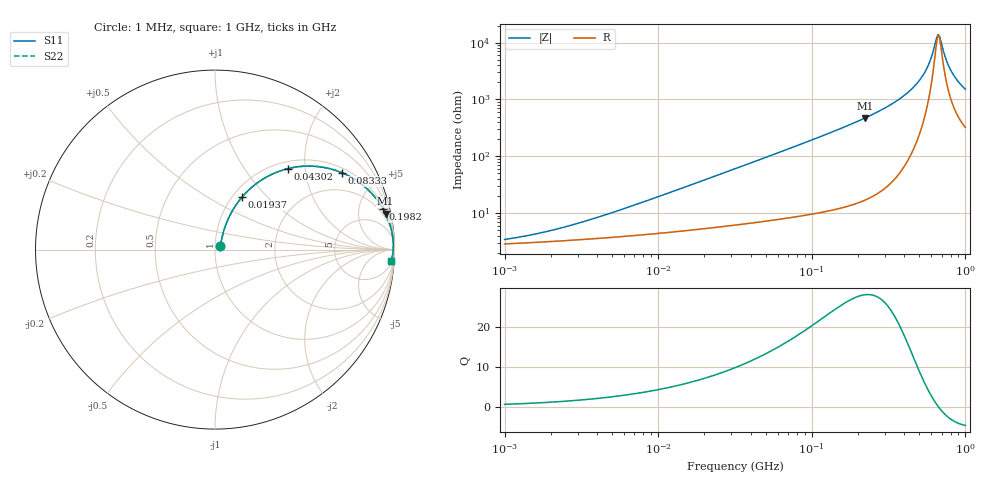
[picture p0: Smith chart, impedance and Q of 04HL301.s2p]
! Coilcraft 0402HL-301 Chip Inductor
! 20 July 2012
# MHz S MA R 50
!Freq  MagS11  AngS11  MagS21  AngS21  MagS12  AngS12  MagS22  AngS22
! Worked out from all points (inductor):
!   304 points, 1 MHz to 1 GHz, reference 50 ohm
!   read as one part in series: L = 300 nH near 6.196 MHz
!   highest Q = 28 at 222.1 MHz (marker M1), where L = 337 nH
!   self-resonance near 663.4 MHz
!   S11 on the Smith chart (normalised r, x): 1 MHz: 1.06, +0.04; 19.37 MHz: 1.10, +0.73; 43.02 MHz: 1.14, +1.63; 83.33 MHz: 1.18, +3.19; 198.2 MHz: 1.30, +8.19; 1 GHz: 7, -29
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1  0.03322 32.4  0.9721 -1.0  0.9721 -1.0  0.03322 32.4
1.768173  0.04401 45.4  0.9696 -1.9  0.9696 -1.9  0.04401 45.4
3.19853  0.06684 57.2  0.9655 -3.3  0.9655 -3.3  0.06684 57.2
10  0.1825 66.7  0.9429 -10.2  0.9429 -10.2  0.1825 66.7
19.36996  0.3314 62.7  0.8977 -19.1  0.8977 -19.1  0.3314 62.7
31.9853  0.4973 54.6  0.8188 -29.7  0.8188 -29.7  0.4973 54.6
43.0193  0.6085 47.9  0.7447 -37.3  0.7447 -37.3  0.6085 47.9
83.32822  0.8275 31.1  0.5179 -55.7  0.5179 -55.7  0.8275 31.1
102.306  0.8753 26.2  0.4427 -61.0  0.4427 -61.0  0.8753 26.2
198.1663  0.9635 13.6  0.235 -74.3  0.235 -74.3  0.9635 13.6
222.0929  0.9712 11.9  0.2062 -76.1  0.2062 -76.1  0.9712 11.9
319.853  0.9869 7.2  0.1261 -80.4  0.1261 -80.4  0.9869 7.2
420.4965  0.9924 4.3  0.07559 -82.1  0.07559 -82.1  0.9924 4.3
516.2633  0.9939 2.4  0.04139 -80.3  0.04139 -80.3  0.9939 2.4
552.8079  0.9939 1.7  0.03054 -77.7  0.03054 -77.7  0.9939 1.7
591.9394  0.9938 1.1  0.02007 -71.3  0.02007 -71.3  0.9938 1.1
663.4103  0.993 0.1  0.007127 -9.5  0.007127 -9.5  0.993 0.1
678.7083  0.9927 -0.1  0.00764 18.0  0.00764 18.0  0.9927 -0.1
743.5105  0.9915 -1.0  0.01862 62.4  0.01862 62.4  0.9915 -1.0
796.1412  0.9903 -1.6  0.02891 69.6  0.02891 69.6  0.9903 -1.6
872.1558  0.9883 -2.4  0.04317 73.0  0.04317 73.0  0.9883 -2.4
1000  0.9841 -3.7  0.06524 74.1  0.06524 74.1  0.9841 -3.7
